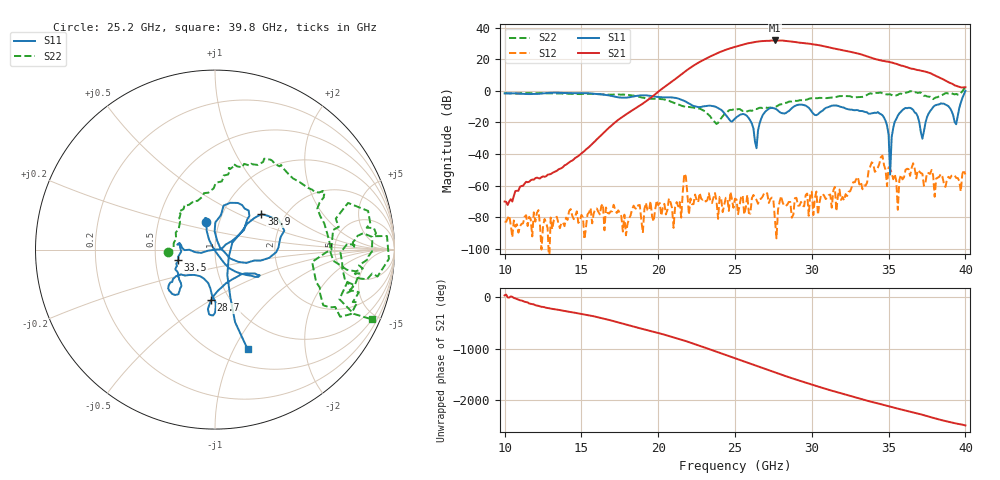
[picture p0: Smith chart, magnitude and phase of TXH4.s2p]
!Keysight Technologies,M9808A,MY58100618,A.14.70.03
!Date: Monday, February 27, 2023 13:37:09
!Correction: S11(C  2-Port  )
!S21(C  2-Port  )
!S12(C  2-Port  )
!S22(C  2-Port  )
!S2P File: Measurements: S11, S21, S12, S22:
# Hz S  RI  R 50
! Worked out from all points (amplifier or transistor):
!   301 points, 10 GHz to 40 GHz, reference 50 ohm
!   highest |S21| = 31.8 dB at 27.6 GHz (marker M1)
!   |S21| within 3 dB of that: 25.38 GHz to 30.47 GHz (5.09 GHz wide, 18.2 % of centre)
!   unconditionally stable (mu >= 1): start of sweep to 39.83 GHz
!   at 15 GHz: K = 41683.44, MAG = -29.8 dB, |S12| = -78.4 dB
!   at 25 GHz: K = 47.55, MAG = 28.2 dB, |S12| = -68.1 dB
!   at 40 GHz: K = -1.10, MSG = 27.6 dB, |S12| = -52.9 dB
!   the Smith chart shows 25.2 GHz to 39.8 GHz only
!   S11 on the Smith chart (normalised r, x): 25.2 GHz: 0.87, +0.27; 28.7 GHz: 0.82, -0.50; 33.5 GHz: 0.66, -0.08; 38.9 GHz: 1.52, +0.67; 39.8 GHz: 0.67, -1.14
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1e10  0.7576 0.3336  0.000252 0.000193  6.29e-05 -3.74e-05  -0.0107 0.8493
1.5e10  0.6108 -0.5845  0.00839 0.00629  5.26e-05 0.000108  0.7408 0.2887
2e10  -0.1631 -0.6157  0.8301 0.4246  -0.000241 3.46e-05  0.2838 -0.4842
2.34e10  -0.3385 -0.0102  5.617 10.88  0.000107 0.000301  0.00747 -0.1531
2.42e10  -0.2227 -0.0313  16.94 -6.68  -5.05e-05 0.000138  -0.1558 -0.0255
2.5e10  -0.0645 0.1149  -6.992 -23.48  -0.000379 0.0001  -0.2666 -0.0256
2.52e10  -0.0491 0.1515  -15.93 -20.57  3.7e-05 -0.000121  -0.2641 -0.0138
2.59e10  -0.0473 0.127  -29.73 12.01  -0.000125 5.53e-05  -0.2181 0.0857
2.65e10  0.0302 -0.0471  -2.125 36  -0.000182 -0.000199  -0.1918 0.2001
2.71e10  0.2023 -0.1457  32.75 18.72  0.00027 -0.000501  -0.1443 0.25
2.76e10  0.2348 -0.1403  35.91 -15.23  2.43e-05 8.42e-05  -0.0609 0.3147
2.81e10  0.1223 -0.1517  9.984 -37.38  -0.000277 -0.000118  0.0374 0.3795
2.87e10  -0.0217 -0.2821  -25.94 -24.86  -9.31e-05 2.95e-05  0.0861 0.4505
2.93e10  -0.011 -0.367  -31.94 7.398  0.000305 -5.36e-05  0.1695 0.4754
3e10  -0.0263 -0.2151  -5.214 29.31  -7.75e-05 -0.00065  0.2912 0.5049
3.09e10  -0.2343 -0.1646  23.89 6.988  0.000137 0.000356  0.4103 0.4197
3.19e10  -0.2006 -0.2364  6.493 -18.46  -0.000261 -0.000242  0.5983 0.3226
3.35e10  -0.2046 -0.0589  -11.41 5.63  0.000625 -0.000788  0.6928 -0.0836
3.5e10  -0.0412 -0.00672  6.467 5.192  -0.000116 0.00381  0.7717 0.00785
3.89e10  0.2585 0.1977  -0.139 1.876  -0.00103 -0.00162  0.7674 -0.2921
3.98e10  0.1824 -0.5563  0.9966 0.7954  0.000191 0.00233  0.8746 -0.3891
4e10  0.4475 -0.8953  1.193 0.5112  -0.00105 -0.00201  1.254 -0.5902
